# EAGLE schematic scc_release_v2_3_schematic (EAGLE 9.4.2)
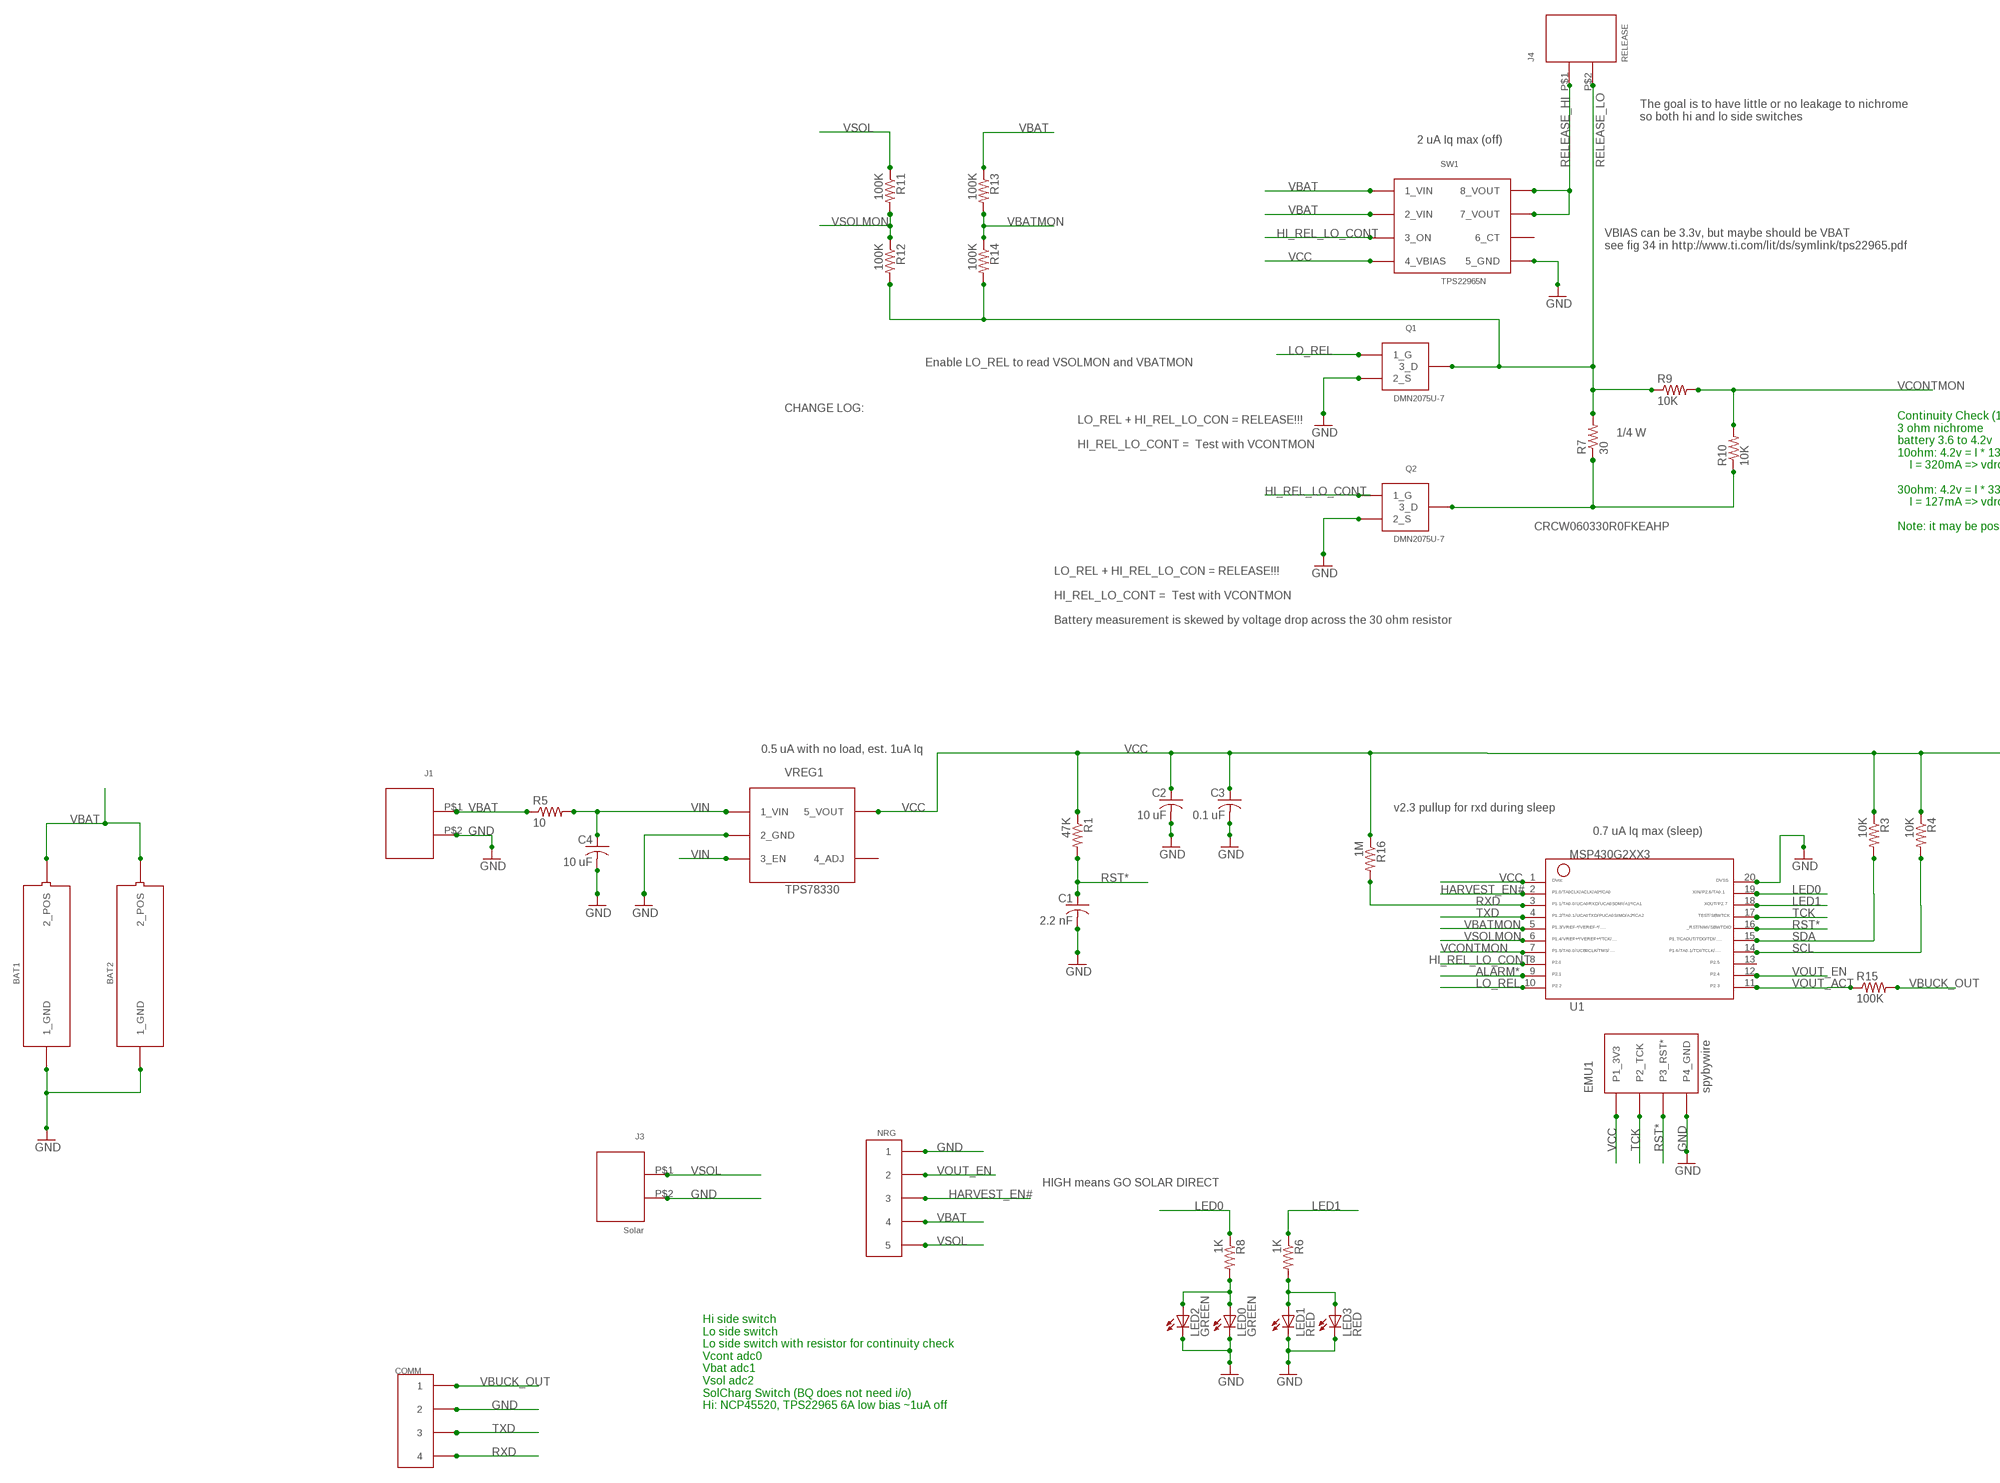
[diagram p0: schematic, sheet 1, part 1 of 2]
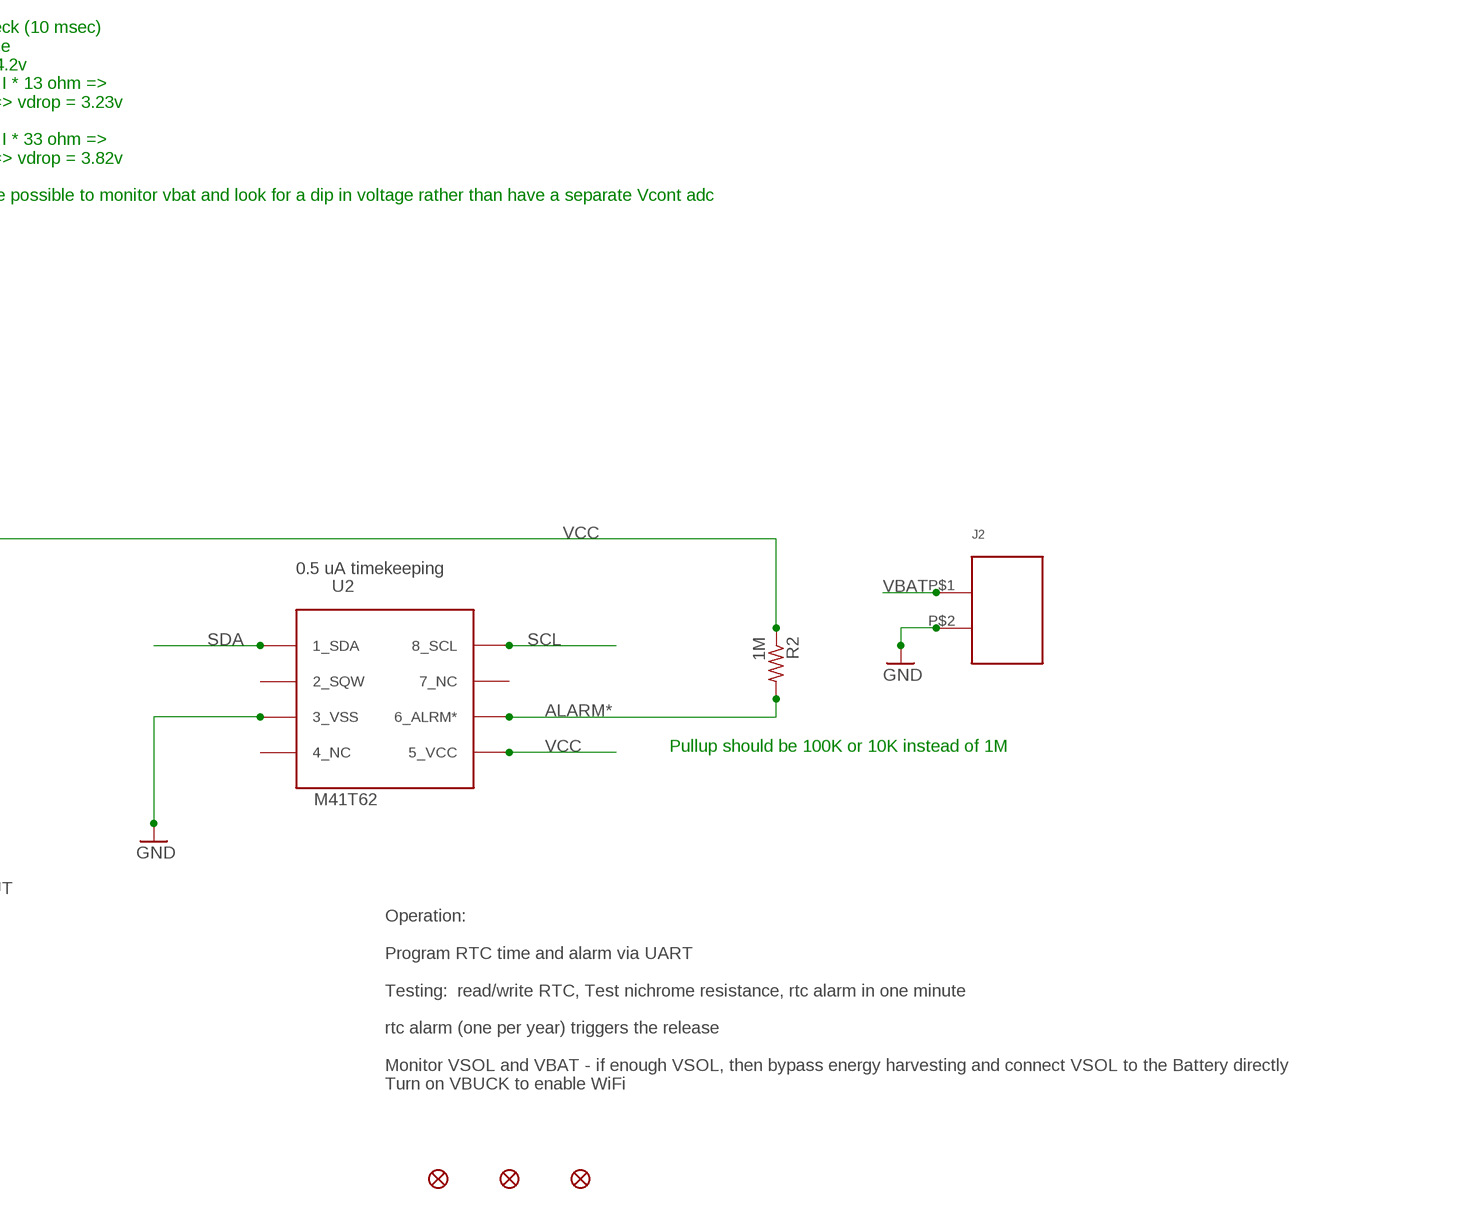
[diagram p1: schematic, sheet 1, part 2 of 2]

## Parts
BAT1  BAT_10440  [BAT_10440]
BAT2  BAT_10440  [BAT_10440]
C1  2.2 nF  C-USC0603K  [C0603K]
C2  10 uF  C-USC0603K  [C0603K]
C3  0.1 uF  C-USC0603K  [C0603K]
C4  10 uF  C-USC0603K  [C0603K]
COMM  CON_1X4_050  [CON_1X4_050]
EMU1  spybywire  EMU_MSP_SPYBYWIRE_4_050  [EMU_MSP_SPYBYWIRE_4_050]
J1  CON_1X2_0_1  [CON_1X2_0_1]
J2  CON_1X2_0_1  [CON_1X2_0_1]
J3  Solar  CON_1X2_0_1  [CON_1X2_0_1]
J4  RELEASE  CON_1X2_0_1  [CON_1X2_0_1]
JP1  FIDUCIAL1.5X3  [FIDUCIAL-1.5X3]
JP2  FIDUCIAL1.5X3  [FIDUCIAL-1.5X3]
JP3  FIDUCIAL1.5X3  [FIDUCIAL-1.5X3]
LED0  GREEN  LEDCHIPLED_0805  [CHIPLED_0805]
LED1  RED  LEDCHIPLED_0805  [CHIPLED_0805]
LED2  GREEN  LEDCHIPLED_0805  [CHIPLED_0805]
LED3  RED  LEDCHIPLED_0805  [CHIPLED_0805]
NRG  CON_1X5_050  [CON_1X5_050]
Q1  DMN2075U-7  FET_A03414  [SOT23-3]
Q2  DMN2075U-7  FET_A03414  [SOT23-3]
R1  47K  R-US_R0603  [R0603]
R2  1M  R-US_R0603  [R0603]
R3  10K  R-US_R0603  [R0603]
R4  10K  R-US_R0603  [R0603]
R5  10  R-US_R0603  [R0603]
R6  1K  R-US_R0603  [R0603]
R7  30  R-US_R0603  [R0603]
R8  1K  R-US_R0603  [R0603]
R9  10K  R-US_R0603  [R0603]
R10  10K  R-US_R0603  [R0603]
R11  100K  R-US_R0603  [R0603]
R12  100K  R-US_R0603  [R0603]
R13  100K  R-US_R0603  [R0603]
R14  100K  R-US_R0603  [R0603]
R15  100K  R-US_R0603  [R0603]
R16  1M  R-US_R0603  [R0603]
SW1  TPS22965N  TPS22965_HISIDESW  [TI_WSON8]
U1  MSP430G2553  G2XX3---PW20  [PW20]
U2  M41T62  [M41T62_PKG]
VREG1  TPS78330  REG101  [SOT23-5]

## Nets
ALARM*: R2.2 U1.9 U2.P$6(6_ALRM*)
GND: BAT1.P$1(1_GND) BAT2.P$1(1_GND) C1.2 C2.2 C3.2 C4.2 COMM.P$2 COMM.P$6 COMM.P$10 EMU1.P4_GND J1.P$2 J2.P$2 J3.P$2 LED0.C LED1.C LED2.C LED3.C NRG.P$1 NRG.P$6 NRG.P$11 Q1.2(2_S) Q2.2(2_S) SW1.P$5(5_GND) SW1.P$9(5_GND) U1.20 U2.P$3(3_VSS) VREG1.P$2(2_GND)
HARVEST_EN#: NRG.P$3 NRG.P$8 NRG.P$13 U1.2
HI_REL_LO_CONT: Q2.1(1_G) SW1.P$3(3_ON) U1.8
LED0: R8.1 U1.19
LED1: R6.1 U1.18
LO_REL: Q1.1(1_G) U1.10
N$1: LED1.A LED3.A R6.2
N$4: Q2.3(3_D) R7.1 R10.1
N$19: LED0.A LED2.A R8.2
RELEASE_HI: J4.P$1 SW1.P$7(7_VOUT) SW1.P$8(8_VOUT)
RELEASE_LO: J4.P$2 Q1.3(3_D) R7.2 R9.1 R12.2 R14.2
RST*: C1.1 EMU1.P3_RST* R1.2 U1.16
RXD: COMM.P$4 COMM.P$8 COMM.P$12 R16.2 U1.3
SCL: R4.2 U1.14 U2.P$8(8_SCL)
SDA: R3.2 U1.15 U2.P$1(1_SDA)
TCK: EMU1.P2_TST(P2_TCK) U1.17
TXD: COMM.P$3 COMM.P$7 COMM.P$11 U1.4
VBAT: BAT1.P$2(2_POS) BAT2.P$2(2_POS) J1.P$1 J2.P$1 NRG.P$4 NRG.P$9 NRG.P$14 R5.1 R13.1 SW1.P$1(1_VIN) SW1.P$2(2_VIN)
VBATMON: R13.2 R14.1 U1.5
VBUCK_OUT: COMM.P$1 COMM.P$5 COMM.P$9 R15.2
VCC: C2.1 C3.1 EMU1.P1_3V3 R1.1 R2.1 R3.1 R4.1 R16.1 SW1.P$4(4_VBIAS) U1.1 U2.P$5(5_VCC) VREG1.P$5(5_VOUT)
VCONTMON: R9.2 R10.2 U1.7
VIN: C4.1 R5.2 VREG1.P$1(1_VIN) VREG1.P$3(3_EN)
VOUT_ACT: R15.1 U1.11
VOUT_EN: NRG.P$2 NRG.P$7 NRG.P$12 U1.12
VSOL: J3.P$1 NRG.P$5 NRG.P$10 NRG.P$15 R11.1
VSOLMON: R11.2 R12.1 U1.6
Unconnected: SW1.P$6(6_CT) U1.13 U2.P$2(2_SQW) U2.P$4(4_NC) U2.P$7(7_NC) VREG1.P$4(4_ADJ)

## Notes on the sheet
- The goal is to have little or no leakage to nichrome
  so both hi and lo side switches
- 2 uA Iq max (off)
- VBIAS can be 3.3v, but maybe should be VBAT
  see fig 34 in http://www.ti.com/lit/ds/symlink/tps22965.pdf
- Enable LO_REL to read VSOLMON and VBATMON
- CHANGE LOG: | 1/4 W
- LO_REL + HI_REL_LO_CON = RELEASE!!!
  
  HI_REL_LO_CONT =  Test with VCONTMON
- CRCW060330R0FKEAHP
- Continuity Check (10 msec)
  3 ohm nichrome
  battery 3.6 to 4.2v
  10ohm: 4.2v = I * 13 ohm =>
      I = 320mA => vdrop = 3.23v 
  
  30ohm: 4.2v = I * 33 ohm =>
      I = 127mA => vdrop = 3.82v 
  
  Note: it may be possible to monitor vbat and look for a dip in voltage rather than have a separate Vcont adc
- LO_REL + HI_REL_LO_CON = RELEASE!!!
  
  HI_REL_LO_CONT =  Test with VCONTMON
  
  Battery measurement is skewed by voltage drop across the 30 ohm resistor
- 0.5 uA with no load, est. 1uA Iq
- 0.5 uA timekeeping
- v2.3 pullup for rxd during sleep
- 0.7 uA Iq max (sleep)
- Pullup should be 100K or 10K instead of 1M
- Operation:
  
  Program RTC time and alarm via UART
  
  Testing:  read/write RTC, Test nichrome resistance, rtc alarm in one minute
  
  rtc alarm (one per year) triggers the release
  
  Monitor VSOL and VBAT - if enough VSOL, then bypass energy harvesting and connect VSOL to the Battery directly
  Turn on VBUCK to enable WiFi
- HIGH means GO SOLAR DIRECT
- Hi side switch
  Lo side switch
  Lo side switch with resistor for continuity check
  Vcont adc0
  Vbat adc1
  Vsol adc2
  SolCharg Switch (BQ does not need i/o)
  Hi: NCP45520, TPS22965 6A low bias ~1uA off

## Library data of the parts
BAT1 BAT2 = ti_thom:BAT_10440
C1-C4 = resistor:C-US: CAPACITOR, American symbol
COMM = thomz:CON_1X4_050
EMU1 = ti_thom:EMU_MSP_SPYBYWIRE_4_050
J1-J4 = thomz:CON_1X2_0_1
JP1-JP3 = EM-shield-V1.0A:FIDUCIAL: Fiducial Alignment Points
LED0 LED1-LED3 = led:LED: LED
NRG = thomz:CON_1X5_050
Q1 Q2 = thomz:FET_A03414
R1-R16 = resistor:R-US_: RESISTOR, American symbol
SW1 = ti_thom:TPS22965_HISIDESW
U1 = TI_MSP430_v16:G2XX3---PW20: MSP430G2XX1 TSSOP (PW) 20 Pin Package
U2 = thomz_rtc:M41T62: STMicro M41T62 RTC with embedded 32.768 xtal, 4.4v tolerant, 350nA timekeeping
VREG1 = thomz:REG101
